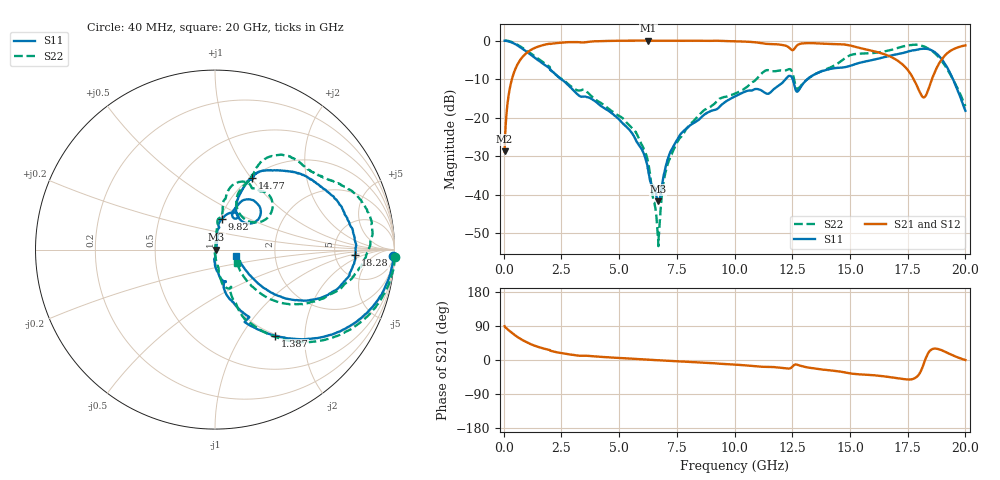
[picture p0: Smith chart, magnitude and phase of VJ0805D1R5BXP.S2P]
! VJ0805D1R5BXP
! DATE 10/29/2021  09:40
! CAPACITORS MOUNTED IN SERIES ON 25 MIL THICK MICROSTRIP SUBSTRATE
# GHz  S  MA  R  50.00
!  FREQ  S11M  S11A  S21M  S21A  S12M  S12A  S22M  S22A
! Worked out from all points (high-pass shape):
!   1601 points, 40 MHz to 20 GHz, reference 50 ohm
!   highest |S21| = 0.02 dB at 6.265 GHz (marker M1); lowest = -28.7 dB at 40 MHz (marker M2)
!   |S21| within 3 dB of the highest: 1.039 GHz to 16.18 GHz (15.14 GHz wide, 176 % of centre); 19.27 GHz to end of sweep
!   lowest |S11| = -41.6 dB at 6.689 GHz (marker M3), VSWR 1.02, Z = 50.8 + j0.000471 ohm
!   |S11| at or under -10 dB: 2.48 GHz to 12.21 GHz (9.728 GHz wide, 132 % of centre); 12.52 GHz to 13.16 GHz (636.5 MHz wide, 4.96 % of centre); 19.46 GHz to end of sweep
!   |S22| runs from -53.3 to 0.0 dB; largest |S21 - S12| = 0.0047
!   S11 on the Smith chart (normalised r, x): 40 MHz: 10, -53; 1.387 GHz: 0.98, -1.43; 9.82 GHz: 1.02, +0.36; 14.77 GHz: 1.01, +1.02; 18.28 GHz: 7.95, -1.25; 20 GHz: 1.27, -0.08
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0.04  0.9934 -2.1  0.03654 89.4  0.0374 88.2  1.004 -2.3
0.21465  0.9751 -11.1  0.1961 78.6  0.1963 78.5  0.9875 -11.4
0.4392  0.9202 -22.1  0.3801 68.0  0.3799 68.0  0.934 -22.6
1.3873  0.5866 -55.0  0.813 36.7  0.8121 36.7  0.6139 -53.8
3.370825  0.1869 -72.3  0.9462 11.1  0.9461 11.1  0.2289 -67.0
5.4292  0.07064 -91.4  0.9966 3.9  0.9961 3.9  0.08004 -80.1
6.265025  0.02034 -85.3  1.002 0.9  1 0.8  0.02587 -92.4
6.689175  0.008286 0.0  0.995 -0.5  0.9948 -0.5  0.002719 -2.5
6.70165  0.00831 5.4  0.9948 -0.6  0.9948 -0.6  0.002164 20.7
7.013525  0.02304 67.7  0.9956 -1.7  0.9941 -1.6  0.02006 84.1
7.512525  0.05159 78.3  0.9945 -3.4  0.9943 -3.4  0.0479 84.5
9.8204  0.1758 77.4  0.9813 -11.5  0.9796 -11.5  0.1955 78.3
10.02  0.1888 74.8  0.9772 -12.2  0.9775 -12.2  0.2058 78.6
11.39225  0.205 57.2  0.9061 -18.1  0.9058 -18.2  0.4135 65.8
12.3653  0.3487 50.9  0.8086 -22.4  0.8088 -22.5  0.4263 47.0
12.63975  0.2333 38.5  0.8191 -11.8  0.8196 -12.0  0.2629 35.3
13.35083  0.3486 65.6  0.926 -21.5  0.925 -21.5  0.3467 67.5
14.77298  0.4506 62.5  0.8891 -32.7  0.889 -32.8  0.5896 60.3
16.68165  0.6304 42.5  0.632 -44.9  0.632 -44.9  0.7434 31.6
18.27845  0.7814 -2.2  0.1926 3.9  0.1923 3.7  0.8223 -6.0
18.98953  0.5687 -30.0  0.5792 25.4  0.578 25.5  0.5377 -34.3
20  0.1231 -15.6  0.8657 -0.0  0.8652 -0.1  0.1413 -30.6
